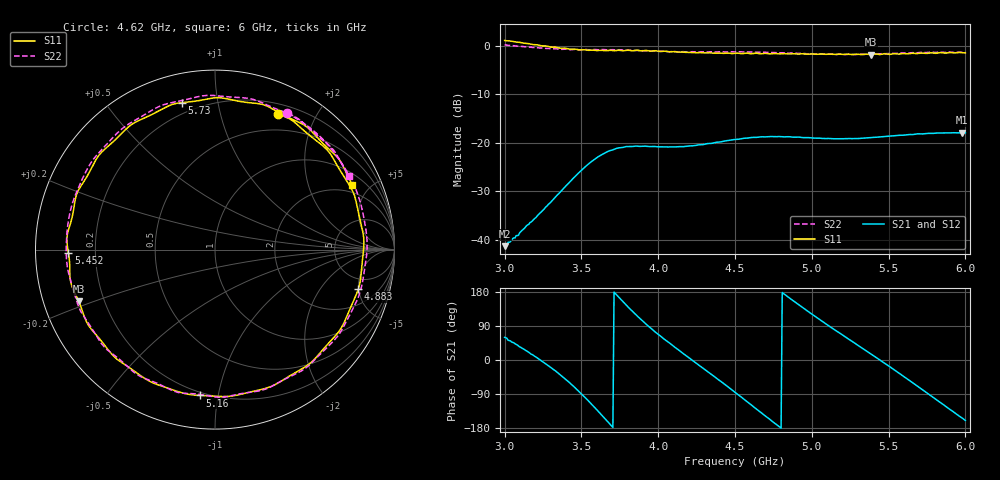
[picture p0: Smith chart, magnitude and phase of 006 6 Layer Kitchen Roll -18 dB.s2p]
!  04/11/2025  14:40:50
! Ref Plane: 0.000 mm
# MHZ S MA R  50
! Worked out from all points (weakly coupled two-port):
!   401 points, 3 GHz to 6 GHz, reference 50 ohm
!   highest |S21| = -17.91 dB at 5.978 GHz (marker M1); lowest = -41.3 dB at 3 GHz (marker M2)
!   lowest |S11| = -1.8 dB at 5.385 GHz (marker M3), VSWR 9.63, Z = 5.36 - j9.09 ohm
!   |S11| at or under -10 dB: nowhere
!   |S22| runs from -1.8 to 0.2 dB; largest |S21 - S12| = 0.0025
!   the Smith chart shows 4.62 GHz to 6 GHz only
!   S11 on the Smith chart (normalised r, x): 4.62 GHz: 0.31, +1.53; 4.883 GHz: 3.54, -4.95; 5.16 GHz: 0.18, -0.89; 5.452 GHz: 0.10, -0.01; 5.73 GHz: 0.14, +0.79; 6 GHz: 1.54, +3.89
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3000  1.136 -112.2  0.008605 59.7  0.008638 61.0  1.023 -115.5
3270  0.9961 179.8  0.02196 -10.5  0.02179 -8.9  0.942 176.8
3390  0.9463 142.0  0.03474 -48.2  0.03492 -47.8  0.9227 138.5
3502.5  0.9112 99.4  0.05249 -90.2  0.05259 -89.8  0.9111 96.0
3607.5  0.8939 54.4  0.0716 -134.4  0.07176 -134.1  0.9087 52.3
3735  0.898 -3.0  0.08821 169.0  0.08863 170.1  0.9082 -2.8
3862.5  0.8998 -55.5  0.09247 116.4  0.09322 117.7  0.8964 -53.7
4005  0.8765 -105.4  0.09102 66.4  0.09088 67.1  0.8771 -103.1
4245  0.8495 -179.6  0.09407 -7.6  0.09456 -6.6  0.8633 -178.1
4357.5  0.8407 146.8  0.09947 -41.2  0.09996 -40.1  0.8673 146.9
4500  0.8379 102.5  0.1083 -85.4  0.1091 -84.6  0.8641 101.1
4620  0.8331 64.9  0.1139 -123.2  0.1141 -122.6  0.8619 62.4
4755  0.8332 23.1  0.1155 -165.9  0.116 -165.1  0.8518 19.0
4882.5  0.8283 -15.4  0.1143 155.3  0.1143 156.0  0.84 -19.7
5002.5  0.8254 -50.8  0.1121 120.5  0.1122 121.1  0.8296 -54.5
5160  0.8169 -95.9  0.1102 76.6  0.1104 77.2  0.8126 -99.0
5385  0.8119 -159.2  0.1131 16.0  0.1136 16.8  0.8227 -158.9
5452.5  0.8165 -178.6  0.1154 -2.6  0.1161 -1.9  0.8292 -177.6
5505  0.8161 167.0  0.1172 -16.9  0.1179 -16.1  0.833 168.0
5730  0.839 102.6  0.1239 -81.2  0.1244 -80.2  0.8526 105.5
5977.5  0.8508 32.4  0.1272 -152.7  0.128 -151.9  0.856 36.0
6000  0.8459 25.2  0.1268 -159.7  0.1274 -159.0  0.8511 28.8
